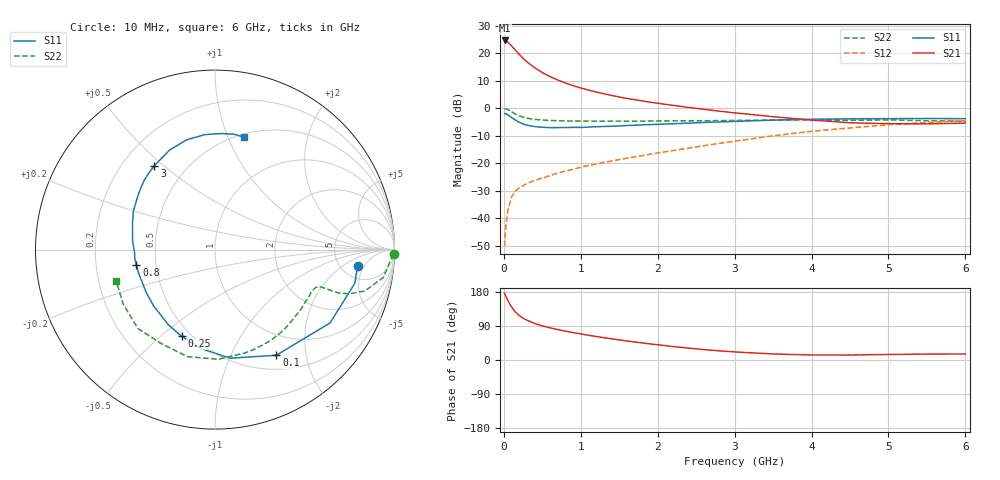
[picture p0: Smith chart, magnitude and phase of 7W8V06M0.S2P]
! Infineon Technologies  Discrete & RF Semiconductors
! BFS17W
! Si NPN RF Bipolar Junction Transistor in SOT323
! VCE = 8 V  IC = 6 mA
! Common Emitter S-Parameters:  August  1999
# GHz  S  MA  R  50
!  f  S11  S21  S12  S22
! GHz  MAG  ANG  MAG  ANG  MAG  ANG  MAG  ANG
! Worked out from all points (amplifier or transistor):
!   36 points, 10 MHz to 6 GHz, reference 50 ohm
!   highest |S21| = 24.7 dB at 10 MHz (marker M1)
!   |S21| within 3 dB of that: start of sweep to 133.6 MHz
!   unconditionally stable (mu >= 1): 537.9 MHz to 2.308 GHz; 5.289 GHz to end of sweep
!   at 250 MHz: K = 0.63, MSG = 23.2 dB, |S12| = -28.2 dB
!   at 1.4 GHz: K = 1.19, MAG = 9.3 dB, |S12| = -19.2 dB
!   at 6 GHz: K = 1.05, MAG = -1.8 dB, |S12| = -4.5 dB
!   S11 on the Smith chart (normalised r, x): 10 MHz: 7.10, -3.62; 100 MHz: 0.69, -1.51; 250 MHz: 0.45, -0.59; 800 MHz: 0.39, -0.08; 3 GHz: 0.33, +0.47; 6 GHz: 0.53, +1.14
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0.01  0.7995 -6.6  17.13 175.7  0.0031 82.2  0.9951 -1.5
0.02  0.8013 -13.5  16.92 170.7  0.0057 84.7  0.9769 -4.0
0.05  0.7603 -32.5  16.09 157.6  0.0136 75.5  0.9507 -9.4
0.1  0.6807 -59.8  13.71 140.1  0.0244 64.2  0.8654 -15.5
0.15  0.6111 -82.0  11.43 126.7  0.031 56.4  0.7844 -18.3
0.2  0.5569 -98.1  9.576 117.5  0.0359 54.3  0.7287 -19.3
0.25  0.5173 -111.1  8.117 110.4  0.039 51.9  0.6878 -19.4
0.3  0.4935 -121.5  7.006 105.0  0.0429 51.7  0.6618 -19.4
0.4  0.4646 -137.3  5.475 96.4  0.0486 53.0  0.6282 -19.4
0.5  0.4515 -148.2  4.469 90.1  0.0538 55.1  0.6111 -19.7
0.6  0.4442 -156.6  3.765 84.9  0.0596 56.9  0.6011 -20.5
0.8  0.4458 -169.1  2.885 76.1  0.0723 60.2  0.589 -23.1
0.9  0.4496 -173.8  2.581 72.4  0.0775 61.7  0.5851 -24.5
1.1  0.4549 177.3  2.144 65.2  0.0912 64.0  0.583 -28.0
1.3  0.4666 170.1  1.836 58.9  0.1039 65.7  0.5807 -32.1
1.6  0.4858 161.2  1.512 50.2  0.1234 68.0  0.5813 -38.4
2.2  0.5231 145.3  1.129 35.5  0.1702 70.9  0.5904 -52.9
3  0.5768 125.8  0.827 21.3  0.2522 70.5  0.5998 -73.9
3.5  0.6092 114.7  0.703 15.9  0.3155 67.4  0.6113 -88.3
4.5  0.6431 95.1  0.545 13.1  0.439 55.8  0.6031 -119.7
5.5  0.6519 80.8  0.52 15.6  0.5514 42.5  0.5948 -149.3
6  0.6465 75.5  0.537 15.9  0.5951 36.0  0.5773 -162.6
